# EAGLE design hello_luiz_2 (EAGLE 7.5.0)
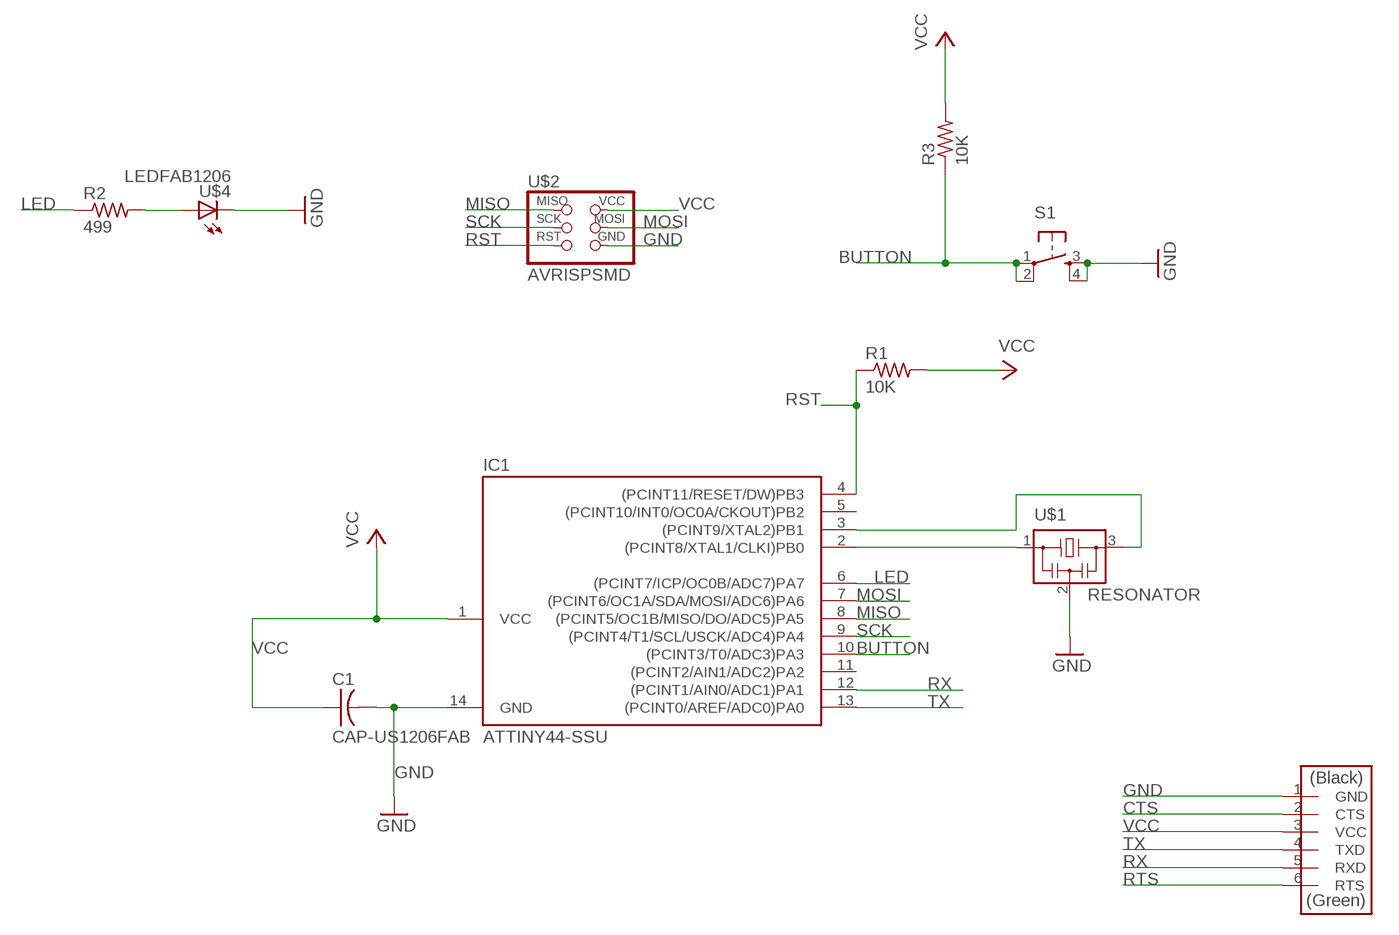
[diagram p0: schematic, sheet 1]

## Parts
C1  CAP-US1206FAB  [C1206FAB]
IC1  ATTINY44-SSU  [SOIC14]
R1  10K  RES-US1206FAB  [R1206FAB]
R2  499  RES-US1206FAB  [R1206FAB]
R3  10K  RES-US1206FAB  [R1206FAB]
S1  6MM_SWITCH6MM_SWITCH  [6MM_SWITCH]
U$1  RESONATOR  [EFOBM]
U$2  AVRISPSMD  [2X03SMD]
U$3  FTDI-SMD-HEADER  [1X06SMD]
U$4  LEDFAB1206  [LED1206FAB]

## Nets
BUTTON: IC1.10((PCINT3/T0/ADC3)PA3) R3.1 S1.1(P) S1.2(P1)
CTS: U$3.2(CTS)
GND: C1.2 IC1.14(GND) S1.3(S) S1.4(S1) U$1.2 U$2.6(GND) U$3.1(GND) U$4.2(C)
LED: IC1.6((PCINT7/ICP/OC0B/ADC7)PA7) R2.1
MISO: IC1.8((PCINT5/OC1B/MISO/DO/ADC5)PA5) U$2.1(MISO)
MOSI: IC1.7((PCINT6/OC1A/SDA/MOSI/ADC6)PA6) U$2.4(MOSI)
N$1: IC1.2((PCINT8/XTAL1/CLKI)PB0) U$1.1
N$2: IC1.3((PCINT9/XTAL2)PB1) U$1.3
N$7: R2.2 U$4.1(A)
RST: IC1.4((PCINT11/RESET/DW)PB3) R1.1 U$2.5(RST)
RTS: U$3.6(RTS)
RX: IC1.12((PCINT1/AIN0/ADC1)PA1) U$3.5(RXD)
SCK: IC1.9((PCINT4/T1/SCL/USCK/ADC4)PA4) U$2.3(SCK)
TX: IC1.13((PCINT0/AREF/ADC0)PA0) U$3.4(TXD)
VCC: C1.1 IC1.1(VCC) R1.2 R3.2 U$2.2(VCC) U$3.3(VCC)
Unconnected: IC1.5((PCINT10/INT0/OC0A/CKOUT)PB2) IC1.11((PCINT2/AIN1/ADC2)PA2)

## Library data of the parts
C1 = fab:CAP-US
IC1 = fab:ATTINY44
R1-R3 = fab:RES-US: Resistor (US Symbol)
S1 = fab:6MM_SWITCH: OMRON SWITCH
U$1 = fab:RESONATOR
U$2 = fab:AVRISP
U$3 = fab:FTDI-SMD-HEADER
U$4 = fab:LED: LED

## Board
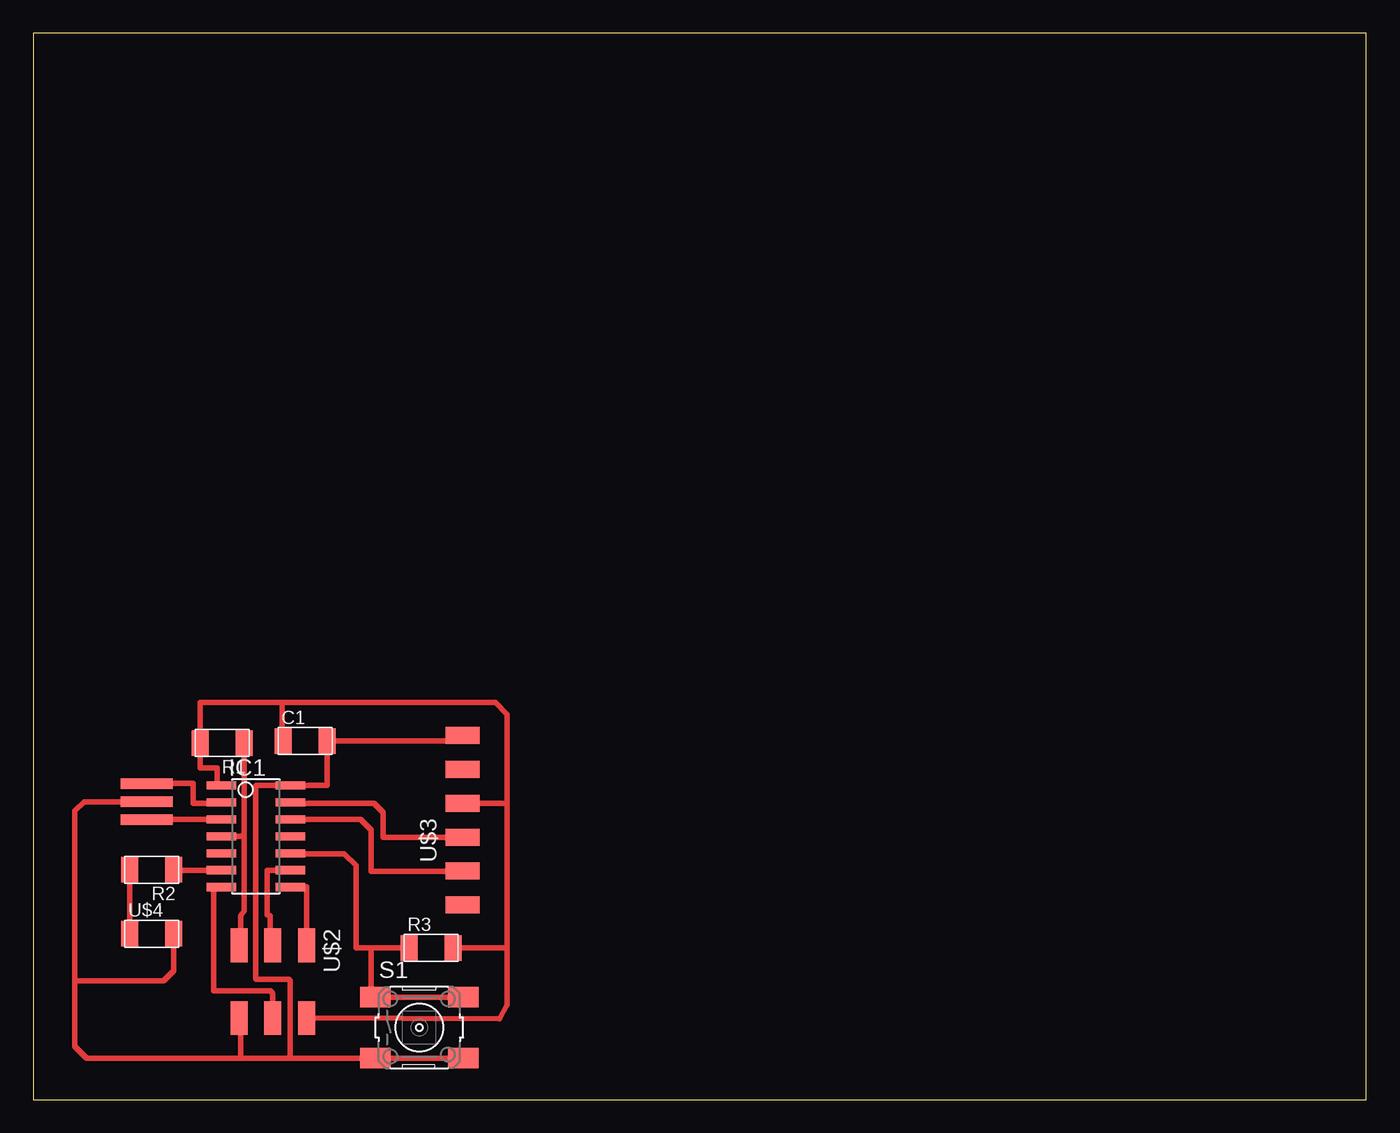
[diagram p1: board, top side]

Size 100 x 80 mm. Coordinates in mm from the lower left corner, seen from the top.
Outline: 0,0 100,0 100,80 0,80 0,0
Copper layers (1*16): Top 0.035mm / dielectric 1.5mm / Bottom 0.035mm
Design rules "default *": minimum track width 10mil, minimum drill 24mil, track to track 16mil, track to pad 16mil, pad to pad 16mil, via to via 16mil, smd to smd 16mil, copper to edge 40mil, drill to drill 8mil, minimum pad ring 10mil, minimum via ring 8mil, stop-mask expansion 4mil, vias tented up to drill 0mil, thermal gap 10mil

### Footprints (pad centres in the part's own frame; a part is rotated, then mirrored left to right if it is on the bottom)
C1206FAB = smd 1.27 x 1.905: 1 -1.651,0; 2 1.651,0
SOIC14 = smd 0.61 x 2.21: 1 -3.81,-2.603; 2 -2.54,-2.603; 3 -1.27,-2.603; 4 0,-2.603; 5 1.27,-2.603; 6 2.54,-2.603; 7 3.81,-2.603; 8 3.81,2.603; 9 2.54,2.603; 10 1.27,2.603; 11 0,2.603; 12 -1.27,2.603; 13 -2.54,2.603; 14 -3.81,2.603
R1206FAB = smd 1.27 x 1.905: 1 -1.651,0; 2 1.651,0
6MM_SWITCH = smd 2.286 x 1.524: 1 -3.302,2.286; 2 3.302,2.286; 3 -3.302,-2.286; 4 3.302,-2.286
EFOBM = smd 0.8 x 3.9: 1 -1.35,0; 2 0,0; 3 1.35,0
2X03SMD = smd 2.54 x 1.27: 1 -2.54,2.54; 2 2.92,2.54; 3 -2.54,0; 4 2.92,0; 5 -2.54,-2.54; 6 2.92,-2.54
1X06SMD = smd 2.54 x 1.27: 1 0,6.35; 2 0,3.81; 3 0,1.27; 4 0,-1.27; 5 0,-3.81; 6 0,-6.35
LED1206FAB = smd 1.27 x 1.905: 1 -1.651,0; 2 1.651,0

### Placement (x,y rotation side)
C1  20.38,26.89 0 top
IC1  16.7,19.75 270 top
R1  14.16,26.75 180 top
R2  8.89,17.24 180 top
R3  29.84,11.37 0 top
S1  28.96,5.4 0 top
U$1  8.51,22.35 270 top
U$2  17.97,9.03 270 top
U$3  32.19,20.95 0 top
U$4  8.89,12.45 0 top

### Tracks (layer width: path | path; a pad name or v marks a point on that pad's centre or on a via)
BUTTON
  Top 0.406: S1.2 S1.1 25.34,7.68 25.34,11.37 | R3.1 25.34,11.37 | 25.34,11.37 24.23,11.37 24.23,17.56 23.34,18.45 19.3,18.45 IC1.10
GND
  Top 0.406: S1.4 S1.3 19.23,3.11 | U$3.1 32.19,26.89 C1.2 22.04,23.56 IC1.14 16.72,23.56 arc90 16.7,23.53 16.7,9.11 arc90 16.81,9 19.17,9 arc-90 19.25,8.92 19.25,3.08 arc90 19.23,3.11 | 19.23,3.11 15.56,3.11 | 15.56,3.11 4,3.11 3.11,4 3.11,8.89 | 3.11,8.89 3.11,21.64 3.81,22.34 8.49,22.34 U$1.2 | U$4.2 10.54,9.65 9.78,8.89 3.11,8.89 | U$2.6 arc-90 15.56,5.99 15.56,3.11
LED
  Top 0.406: IC1.6 10.54,17.21 R2.1
MISO
  Top 0.406: IC1.8 20.51,15.94 U$2.1
MOSI
  Top 0.406: IC1.7 13.53,15.94 13.53,8.17 17.67,8.17 arc-90 17.95,7.89 17.95,6.14 arc90 U$2.4
N$1
  Top 0.406: 14.03,22.23 arc90 IC1.2 14.1,22.23 12,22.23 12,23.7 U$1.1
N$2
  Top 0.406: U$1.3 14.1,21 IC1.3
N$7
  Top 0.406: R2.2 U$4.1
RST
  Top 0.406: R1.1 15.81,20 | 15.81,20 15.81,14.14 15.56,13.78 15.56,11.81 U$2.5 | IC1.4 15.56,19.75 arc90 15.81,20
RX
  Top 0.406: U$3.5 32.19,17.11 25.34,17.11 25.34,20.23 24.54,21.02 IC1.12
SCK
  Top 0.406: 17.78,12.67 U$2.3 17.78,11.57 17.78,13.78 17.56,13.86 17.56,17.2 IC1.9
TX
  Top 0.406: U$3.4 26.23,19.68 26.23,21.56 25.56,22.23 19.3,22.23 IC1.13
VCC
  Top 0.406: 35.56,11.37 35.56,22.23 | C1.1 18.67,26.89 18.67,29.78 | R3.2 35.56,11.37 | U$3.3 35.56,22.23 | 18.67,29.78 12.51,29.78 R1.2 12.51,24.89 13.78,24.89 13.78,23.56 IC1.1 | U$2.2 34.98,6.06 35.56,7.11 35.56,11.37 | 18.67,29.78 34.67,29.78 35.56,28.89 35.56,22.23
